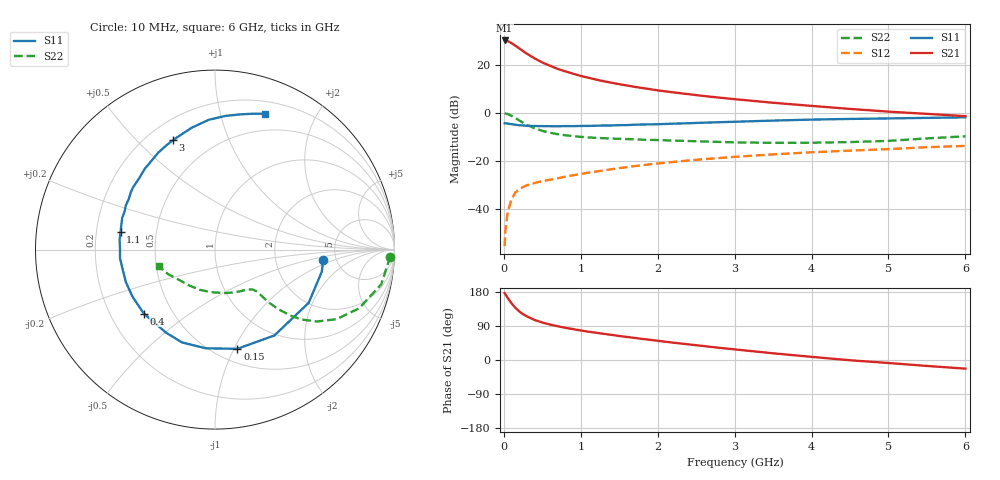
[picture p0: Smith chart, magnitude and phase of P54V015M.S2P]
! SIEMENS Small Signal Semiconductors
! BFP183
! Si NPN RF Bipolar Junction Transistor in SOT143
! VCE = 4 V  IC = 15 mA
! Common Emitter S-Parameters:  March  1996
# GHz  S  MA  R  50
!  f  S11  S21  S12  S22
! GHz  MAG  ANG  MAG  ANG  MAG  ANG  MAG  ANG
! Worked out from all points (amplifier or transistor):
!   36 points, 10 MHz to 6 GHz, reference 50 ohm
!   highest |S21| = 30.1 dB at 10 MHz (marker M1)
!   |S21| within 3 dB of that: start of sweep to 187.3 MHz
!   unconditionally stable (mu >= 1): 974.5 MHz to 5.604 GHz
!   at 250 MHz: K = 0.40, MSG = 28.2 dB, |S12| = -30.8 dB
!   at 1.4 GHz: K = 1.11, MAG = 16.0 dB, |S12| = -23.4 dB
!   at 6 GHz: K = 0.96, MSG = 6.2 dB, |S12| = -13.7 dB
!   S11 on the Smith chart (normalised r, x): 10 MHz: 3.92, -0.75; 150 MHz: 0.63, -1.03; 400 MHz: 0.34, -0.34; 1.1 GHz: 0.31, +0.08; 3 GHz: 0.30, +0.64; 6 GHz: 0.32, +1.39
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0.01  0.6059 -5.7  31.92 176.6  0.0017 86.0  0.9771 -2.3
0.02  0.6076 -11.7  31.7 173.7  0.0036 82.7  0.9662 -4.8
0.05  0.6003 -29.6  31 163.7  0.0088 81.9  0.9462 -11.8
0.1  0.5817 -55.3  28.09 149.5  0.0161 66.2  0.8678 -22.1
0.15  0.5666 -77.3  24.85 137.6  0.0221 60.2  0.7801 -29.8
0.2  0.5523 -95.3  21.88 128.2  0.0259 54.3  0.695 -35.2
0.25  0.549 -109.5  19.1 120.8  0.0288 50.8  0.6226 -38.8
0.3  0.5372 -120.5  16.92 115.1  0.0313 48.8  0.5635 -41.0
0.4  0.5332 -138.0  13.54 105.6  0.0349 46.9  0.4793 -43.4
0.5  0.5292 -150.5  11.13 98.9  0.0381 45.8  0.4234 -44.4
0.6  0.5287 -160.0  9.517 93.5  0.0408 46.2  0.3861 -44.7
0.7  0.5263 -167.8  8.183 89.0  0.0438 46.9  0.3607 -44.8
0.9  0.5293 179.8  6.508 81.5  0.0505 48.2  0.3286 -45.2
1.1  0.5349 169.4  5.358 74.7  0.0573 48.9  0.3083 -46.4
1.5  0.5546 153.6  3.941 63.3  0.0711 49.3  0.2886 -50.4
1.8  0.5734 142.8  3.285 55.6  0.0816 48.6  0.2771 -55.0
2.2  0.596 131.1  2.669 45.8  0.0955 46.3  0.2657 -62.4
3  0.6529 111.2  1.926 28.0  0.1218 40.6  0.2437 -81.4
3.5  0.6906 101.0  1.621 17.7  0.1372 36.7  0.2381 -95.4
4.5  0.7476 85.4  1.208 -0.7  0.1643 28.2  0.2473 -126.9
5.5  0.7864 74.3  0.953 -15.7  0.1934 20.9  0.2947 -152.3
6  0.8073 69.7  0.853 -22.8  0.2058 16.3  0.3263 -163.5
